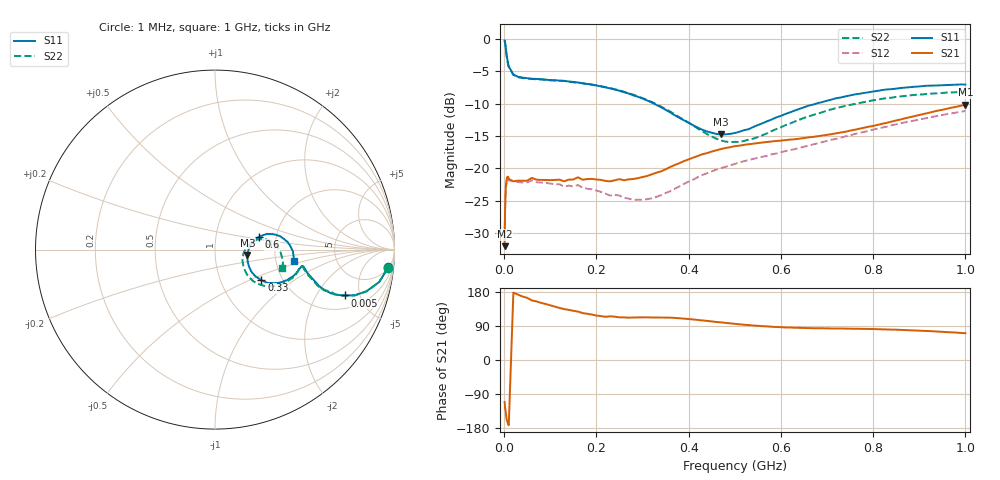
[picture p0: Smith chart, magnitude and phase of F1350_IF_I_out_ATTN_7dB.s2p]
! S-parameters for IF_I+ & IF_I- IDT F1350 DPD Demodulator
! Date Measured:  2015-11-25  RGG
!  Port 1 = Pin 19 = IF_I+
!  Port 2 = Pin 20 = IF_I-
! State: 7 dB attenuation (Gain = Gmax - 7 dB)
! IF Frequency:  1 MHz to 1000 MHz
! RF_INX, RF_INY, IF_Q+, and IF_Q- terminated
! 2300 MHz, 0 dBm signal applied to LO_IN
! Vcc = +5.00 Volts  Icc = approx 275 mA.
! NOTES:  The device was measured on a custom printed circuit evaluation board with individual 50 ohm
!  microstrip lines to the RF and LO pins. The IF outputs are normally connected to balun
!  transformers, which convert the balanced IF output signals to single ended (SE) 50 ohm signals
!  for normal test purposes. For these measurements, to measure the IFI+ and IFI- output SE s-parameters,
!  the chokes associated with the IFI+ and IFI- outputs were removed and a pair of pigtailed
!  50 ohm coaxial lines were soldered to the PCB at these points. 5.00 volt bias was provided
!  to these pins via external bias tees. Data was collected using a calibrated vector
!  network analyzer.  The pigtailed 50 ohm coaxial lines were de-embedded using reference
!  plane extensions. 100 ohm microstrip lines of length 386 mils and 218 mils for the IF_I+ and IF_I-
!  signals, respectively, were de-embedded using Agilent ADS, yielding the reference plane at the IC edge.
!  Only IFI+ and IFI- outputs were measured. IF_Q+ and IF_Q- should be identical.
!  This data is single-ended relative to ports IF_I+ and IF_I- (reference impedance = 50 ohms)
!  Common mode or differential S-parameters may be extracted from this data with a linear simulator.
# mhz S db R 50
! freq  dbS11  angS11  dbS21  angS21  dbS12  angS12  dbS22  angS22
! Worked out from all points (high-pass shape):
!   109 points, 1 MHz to 1 GHz, reference 50 ohm
!   highest |S21| = -10.18 dB at 1 GHz (marker M1); lowest = -32.0 dB at 1 MHz (marker M2)
!   |S21| within 3 dB of the highest: 816 MHz to end of sweep
!   lowest |S11| = -14.8 dB at 470 MHz (marker M3), VSWR 1.45, Z = 71.8 - j4.52 ohm
!   |S11| at or under -10 dB: 324.5 MHz to 676.8 MHz (352.3 MHz wide, 70.4 % of centre)
!   |S22| runs from -15.9 to -0.3 dB; largest |S21 - S12| = 0.066
!   S11 on the Smith chart (normalised r, x): 1 MHz: 5, -18; 5 MHz: 2.90, -3.58; 330 MHz: 1.56, -0.59; 600 MHz: 1.62, +0.25; 1 GHz: 2.52, -0.40
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1  -0.26 -5.8  -32.00 -110.8  -30.85 -105.0  -0.26 -6.1
2  -0.60 -11.1  -26.42 -124.7  -26.06 -116.2  -0.63 -11.3
3  -1.16 -15.4  -24.01 -132.2  -24.08 -130.3  -1.15 -15.5
4  -1.72 -18.1  -22.42 -143.5  -22.63 -143.2  -1.75 -18.2
5  -2.32 -19.5  -21.97 -153.8  -22.61 -151.2  -2.35 -19.7
6  -2.81 -20.4  -21.45 -160.2  -21.82 -158.6  -2.91 -20.4
10  -4.27 -19.1  -21.64 -171.9  -21.87 -171.2  -4.33 -19.4
20  -5.51 -14.1  -21.99 177.8  -21.98 178.0  -5.57 -14.5
40  -6.00 -10.7  -21.90 167.6  -22.19 168.1  -6.06 -11.1
70  -6.19 -11.1  -21.74 154.8  -22.14 156.6  -6.25 -11.6
160  -6.75 -18.9  -21.37 127.7  -22.57 129.2  -6.76 -20.3
170  -6.85 -19.7  -21.74 123.9  -22.98 125.9  -6.87 -20.9
280  -8.73 -30.6  -21.63 112.1  -24.85 115.6  -8.62 -33.5
330  -10.19 -33.4  -20.67 112.2  -24.39 122.8  -10.11 -38.1
340  -10.56 -33.5  -20.46 112.0  -24.13 123.6  -10.46 -38.9
430  -14.04 -22.2  -17.80 104.4  -21.00 123.6  -14.28 -32.5
470  -14.75 -9.6  -17.01 99.4  -19.96 119.7  -15.68 -21.5
510  -14.34 3.3  -16.49 94.3  -19.06 116.0  -15.92 -7.7
600  -11.89 16.2  -15.71 86.7  -17.51 109.1  -13.66 11.0
670  -10.16 16.3  -15.14 83.9  -16.29 104.7  -11.75 13.2
840  -7.77 5.2  -12.77 80.2  -13.34 92.8  -9.09 1.3
1000  -7.06 -8.3  -10.18 70.7  -11.14 78.4  -8.19 -15.0
